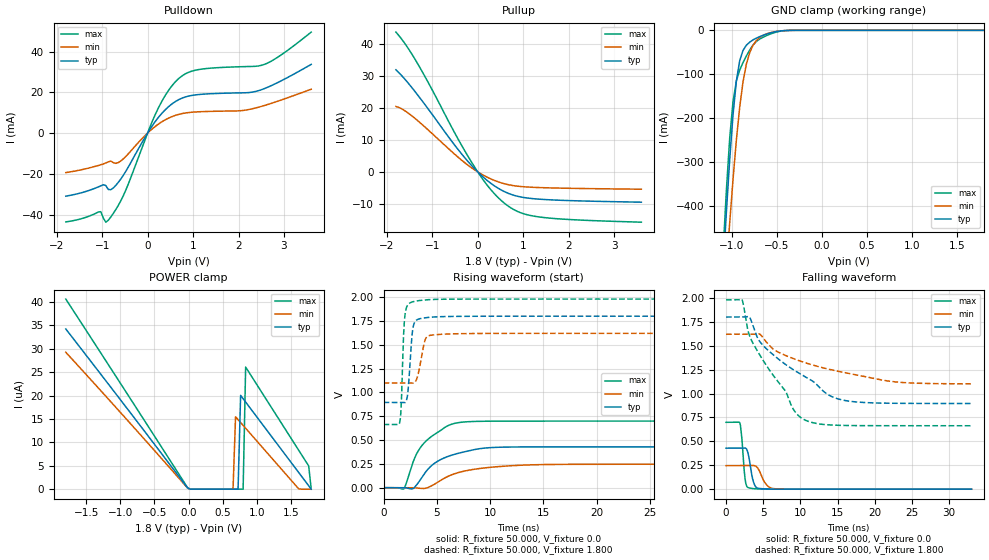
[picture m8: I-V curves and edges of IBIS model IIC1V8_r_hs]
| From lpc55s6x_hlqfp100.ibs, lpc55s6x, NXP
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|   Model IIC1V8_r_hs
[Model] IIC1V8_r_hs
Model_type I/O
Polarity   Non-Inverting
Enable   Active-Low
Vinl =  0.540V
Vinh =  1.260V
Vmeas =  0.900V
Cref =  0.0F
Rref =  100.000
Vref =  0.0V
C_comp   2.515pF   2.512pF   2.535pF
C_comp_pullup   0.454pF   0.388pF   0.547pF
C_comp_pulldown   1.736pF   1.670pF   1.792pF
[Model Spec]
Vinh   1.260V   1.134V   1.386V
Vinl   0.540V   0.486V   0.594V
Vmeas   0.900V   0.810V   0.990V
Vref   0.0V   0.0V   0.0V
Cref   0.0F   0.0F   0.0F
Rref   1000.000   1000.000   1000.000
[Temperature Range]   25.000   0.125k   -40.000
[Voltage Range]   1.800V   1.620V   1.980V
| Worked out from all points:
|   slope of the pulldown table from 0 to 0.27 V, typ, clamps not added: 31.5 ohm
|   slope of the pullup table from 0 to 0.27 V, typ, clamps not added: 79.6 ohm
|   GND clamp passes 1 mA (typ) near -0.44 V on its own axis
|   rising waveform, R_fixture 50.000, V_fixture 0.0: 20-80 % time 2.97ns typ, 3.77ns min, 2.39ns max; typ from 0 V to 0.429 V
|   rising waveform, R_fixture 50.000, V_fixture 1.800: 20-80 % time 347ps typ, 537ps min, 255ps max; typ from 0.895 V to 1.8 V
|   falling waveform, R_fixture 50.000, V_fixture 0.0: 20-80 % time 598ps typ, 964ps min, 409ps max; typ from 0.429 V to 0 V
|   falling waveform, R_fixture 50.000, V_fixture 1.800: 20-80 % time 8.38ns typ, 11.2ns min, 5.72ns max; typ from 1.8 V to 0.896 V
[Pulldown]
|Voltage   I(typ)   I(min)   I(max)
-1.8V     -30.97mA   -19.41mA   -43.61mA
-1.03V    -25.91mA   -15.56mA   -38.59mA
-920mV    -25.75mA   -14.67mA   -43.75mA
-865mV    -27.69mA   -14.16mA   -42.79mA
-700mV    -25.69mA   -14.87mA   -37.58mA
-480mV    -18.8mA    -11.48mA   -28.03mA
235mV     7.619mA    4.356mA    12.23mA
455mV     12.83mA    7.267mA    20.76mA
730mV     16.88mA    9.427mA    27.6mA
1.17V     19mA       10.49mA    31.33mA
2.545V    21.61mA    13.36mA    33.53mA
3.6V      33.71mA    21.52mA    49.57mA
[Pullup]
|Voltage   I(typ)   I(min)   I(max)
-1.8V     32.05mA    20.54mA    43.88mA
-1.57V    28.56mA    18.87mA    39.61mA
-1.295V   23.65mA    15.77mA    33.3mA
-1.02V    18.4mA     12.24mA    26.22mA
-470mV    7.714mA    5.076mA    11.29mA
-30mV     432.2uA    271.3uA    660.2uA
300mV     -3.713mA   -2.28mA    -5.781mA
630mV     -6.475mA   -3.874mA   -10.31mA
960mV     -7.909mA   -4.606mA   -12.9mA
1.4V      -8.61mA    -4.943mA   -14.23mA
2.17V     -9.075mA   -5.188mA   -15.07mA
3.6V      -9.515mA   -5.442mA   -15.79mA
[GND_clamp]
|Voltage   I(typ)   I(min)   I(max)
-1.8V     -3.488A    -3.23A     -3.872A
-1.097V   -545.5mA   -658.5mA   -507mA
-1.06V    -414.6mA   -546.1mA   -365mA
-1.023V   -294.9mA   -439.1mA   -245.9mA
-986mV    -192.4mA   -339.6mA   -162mA
-949mV    -115.6mA   -250.3mA   -115.1mA
-912mV    -69.19mA   -175.2mA   -90.62mA
-838mV    -34.02mA   -77.16mA   -58.5mA
-764mV    -21.82mA   -34.11mA   -33.6mA
-653mV    -11.43mA   -11.65mA   -15.83mA
-431mV    -835.3uA   -879.6uA   -1.141mA
1.8V      0A         0A         0A
[POWER_clamp]
|Voltage   I(typ)   I(min)   I(max)
-1.8V     34.22uA    29.25uA    40.61uA
-13mV     251.2nA    223.3nA    296.4nA
24mV      0A         0A         0A
653mV     0A         0A         0A
690mV     0A         15.47uA    0A
727mV     0A         14.85uA    0A
764mV     20.04uA    14.24uA    0A
801mV     19.32uA    13.62uA    0A
838mV     18.61uA    13.01uA    26.08uA
1.615V    3.579uA    80.87nA    8.337uA
1.763V    715.6nA    0A         4.957uA
1.8V      0A         0A         0A
[Ramp]
| variable   typ   min   max
dV/dt_r   0.257/2.974n   0.148/3.773n   0.419/2.390n
dV/dt_f   0.543/8.379n   0.311/11.175n   0.790/5.718n
R_load = 50.000
[Rising Waveform]
R_fixture= 50.000
V_fixture= 0.0
V_fixture_min= 0.0
V_fixture_max= 0.0
|time   V(typ)   V(min)   V(max)
0s        6.59nV     69.96nV    4.613nV
1.899ns   194.8uV    -158.3nV   -12.49mV
2.78ns    -8.398mV   -69.49uV   273.6mV
3.587ns   107.2mV    -8.163mV   441mV
4.867ns   263mV      42.48mV    565.6mV
6.007ns   326.6mV    116.8mV    649.1mV
6.837ns   355.9mV    152.5mV    679.1mV
9.479ns   415.6mV    207.4mV    697.4mV
13.66ns   428mV      238.9mV    698.9mV
33ns      428.6mV    246.2mV    699.1mV
[Rising Waveform]
R_fixture= 50.000
V_fixture= 1.800
V_fixture_min= 1.620
V_fixture_max= 1.980
|time   V(typ)   V(min)   V(max)
0s        895.1mV    1.1V       663mV
1.514ns   895.1mV    1.1V       686.6mV
1.639ns   895.2mV    1.1V       839.9mV
1.968ns   892.5mV    1.1V       1.775V
2.278ns   1.003V     1.1V       1.921V
2.637ns   1.563V     1.097V     1.948V
2.994ns   1.75V      1.115V     1.958V
3.871ns   1.783V     1.543V     1.972V
4.427ns   1.79V      1.6V       1.975V
33ns      1.8V       1.62V      1.98V
[Falling Waveform]
R_fixture= 50.000
V_fixture= 0.0
V_fixture_min= 0.0
V_fixture_max= 0.0
|time   V(typ)   V(min)   V(max)
0s        428.7mV    246.3mV    699.2mV
1.875ns   428.7mV    246.3mV    688.3mV
2.085ns   428.6mV    246.3mV    571.6mV
2.553ns   430.4mV    246.3mV    110.7mV
3.081ns   331.1mV    246.3mV    13.51mV
3.703ns   72.16mV    247.4mV    5.586mV
4.445ns   7.613mV    197.2mV    2.189mV
5.381ns   2.552mV    51.85mV    818.5uV
6.461ns   979uV      5.202mV    303.6uV
33ns      945.6nV    1.919uV    548.8nV
[Falling Waveform]
R_fixture= 50.000
V_fixture= 1.800
V_fixture_min= 1.620
V_fixture_max= 1.980
|time   V(typ)   V(min)   V(max)
0s        1.8V       1.62V      1.98V
2.133ns   1.8V       1.62V      1.984V
2.933ns   1.806V     1.62V      1.663V
3.544ns   1.727V     1.62V      1.537V
5.115ns   1.492V     1.569V     1.331V
7.983ns   1.305V     1.399V     1.027V
9.254ns   1.239V     1.36V      811.6mV
10.53ns   1.181V     1.325V     726.2mV
16.1ns    925.6mV    1.216V     666.1mV
33ns      895.7mV    1.101V     663.2mV
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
